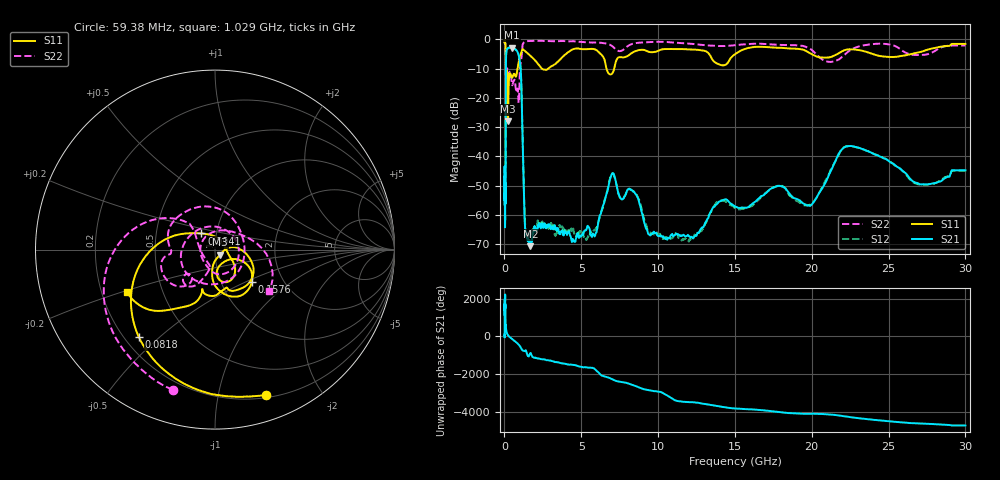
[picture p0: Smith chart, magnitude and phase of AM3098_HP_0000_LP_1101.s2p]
! Date/Time: Thu, Feb 28, 2019 8:31 AM
! Network Analyzer: Agilent Technologies E8364B Rev: A.07.50.67
! Sweep from 0.010 to 30.000 GHz, 1601 Points, Sweep Type: LOG
! Power Supply: 5.022 V, 0.002 A
# Hz S DB R 50
!freq MagS11 AngS11 MagS21 AngS21 MagS12 AngS12 MagS22 AngS22
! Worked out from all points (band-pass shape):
!   1601 points, 10 MHz to 30 GHz, reference 50 ohm
!   highest |S21| = -2.79 dB at 490.6 MHz (marker M1); lowest = -70.7 dB at 1.689 GHz (marker M2)
!   |S21| within 3 dB of the highest: 104.7 MHz to 944.8 MHz (840.2 MHz wide, 160 % of centre)
!   lowest |S11| = -28.0 dB at 231.6 MHz (marker M3), VSWR 1.08, Z = 52.9 - j2.96 ohm
!   |S11| at or under -10 dB: 90.38 MHz to 849.6 MHz (759.3 MHz wide, 162 % of centre); 2.453 GHz to 2.841 GHz (388.5 MHz wide, 14.7 % of centre); 6.642 GHz to 7.141 GHz (498.2 MHz wide, 7.23 % of centre)
!   |S22| runs from -22.8 to -0.4 dB; largest |S21 - S12| = 0.012
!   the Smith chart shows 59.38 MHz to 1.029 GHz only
!   S11 on the Smith chart (normalised r, x): 59.38 MHz: 0.23, -1.39; 81.8 MHz: 0.26, -0.43; 94.1 MHz: 0.85, +0.15; 157.6 MHz: 1.39, -0.54; 1.029 GHz: 0.31, -0.21
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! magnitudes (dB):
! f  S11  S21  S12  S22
! 10 MHz  -0.3  -46.8  -43.4  -0.6
! 38.04 MHz  -0.5  -63.5  -62.5  -1.0
! 59.38 MHz  -1.3  -51.3  -51.3  -1.8
! 71.1 MHz  -2.0  -55.9  -50.8  -2.5
! 81.8 MHz  -3.8  -32.7  -32.9  -4.2
! 94.1 MHz  -18.6  -10.8  -10.8  -21.5
! 144.7 MHz  -14.3  -3.5  -3.4  -12.7
! 157.6 MHz  -11.3  -3.4  -3.3  -10.7
! 231.6 MHz  -28.0  -2.9  -2.9  -12.0
! 490.6 MHz  -13.1  -2.8  -2.8  -15.5
! 550.5 MHz  -12.4  -3.0  -3.0  -14.9
! 926.3 MHz  -7.8  -5.4  -5.3  -21.7
! 1.029 GHz  -5.3  -8.6  -8.6  -8.4
! 1.355 GHz  -4.1  -65.6  -63.9  -0.8
! 1.689 GHz  -5.6  -70.7  -66.3  -0.5
! 2.084 GHz  -7.7  -65.5  -65.2  -0.5
! 5.365 GHz  -3.3  -64.5  -68.0  -1.0
! 7.926 GHz  -5.9  -52.4  -52.5  -2.7
! 11.83 GHz  -3.3  -67.3  -68.3  -1.4
! 19.9 GHz  -4.7  -56.9  -56.5  -3.2
! 22.67 GHz  -3.4  -36.5  -36.6  -3.2
! 30 GHz  -1.5  -44.7  -44.8  -2.1
